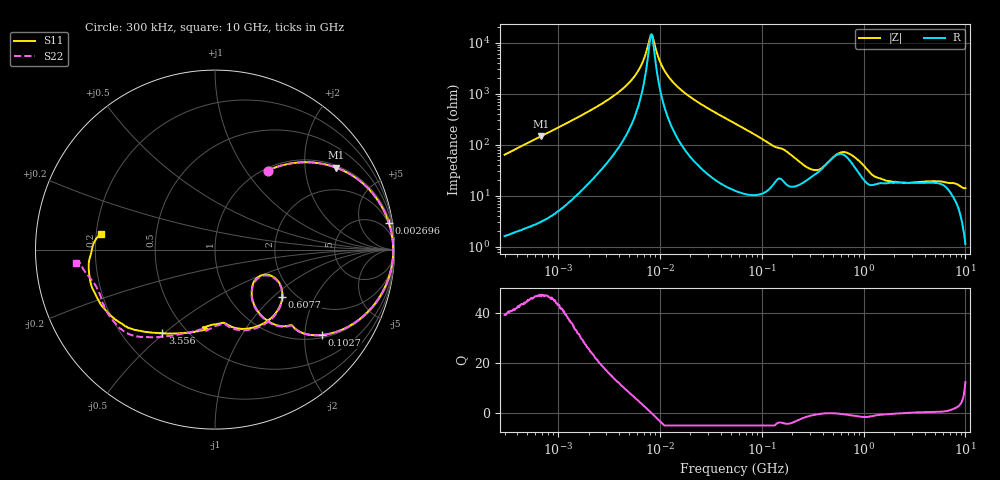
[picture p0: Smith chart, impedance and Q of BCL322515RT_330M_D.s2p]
! S-Parameter Data Generated by TDK Corporation
! Copyright(C) 2024 TDK Corporation.
! All Rights Reserved.
! TDK P/N: BCL322515RT-330M-D (SMD / SMT Inductor (Coil))
! Property: L=33uH at 1MHz
! Size(LxWxT): 3.2x2.5x1.5mm
! Model Type: s2p (Touchstone File Format Version 1.0)
! Frequency: DC=Yes Start=0.3MHz Stop=10000MHz 802points Log-sweep
! Model Generated on May 28, 2024
! Terms and conditions regarding TDK Simulation Models:
! 1)This simulation model is being provided solely for informational
!  purposes. Please refer to the specifications of the products in
!  terms of detailed characteristics of such products.
! 2)In no event shall TDK Corporation of any of its subsidiaries be
!  liable for any loss or damage arising, directly or indirectly,
!  from any information contained in this simulation model, including,
!  but not limited to loss or damages arising from any inaccuracies,
!  omissions or errors in connection with such information.
! 3)Any and all copyrights on this simulation model are owned by
!  TDK Corporation.  Duplication or redistribution of this simulation
!  model without prior written permission from TDK Corporation
!  is prohibited.
! 4)This simulation model is subject to any modification or change
!  without any prior notice.
! 5)Neither TDK Corporation nor any of its subsidiaries shall make any
!  warranty, express or implied, including but not limited to the
!  correctness, implied warranties of merchantability and fitness for
!  a particular purpose with respect to this simulation models.
! 6)The use of this simulation model shall be deemed to have consented
!  to the terms and conditions hereof.
! Port Assignments:
!  1 ---@@@--- 2
! Applicable Conditions:
!  Temperature = 25 degC
!  DC Bias Current = 0 A
!  Small Signal Operation
# Hz S MA R 50
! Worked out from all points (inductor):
!   801 points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, 300 kHz to 10 GHz, reference 50 ohm
!   read as one part in series: L = 33.7 uH near 318.3 kHz
!   highest Q = 47.1 at 680.6 kHz (marker M1), where L = 33.9 uH
!   self-resonance near 8.247 MHz
!   S11 on the Smith chart (normalised r, x): 300 kHz: 1.04, +1.27; 2.696 MHz: 2, +13; 102.7 MHz: 1.08, -2.43; 607.7 MHz: 1.72, -1.14; 3.556 GHz: 0.37, -0.49; 10 GHz: 0.22, +0.06
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300000  0.5287 56.3  0.8348 -32.2  0.8351 -32.1  0.529 56.4
680647  0.8148 34.1  0.5626 -54.7  0.5629 -54.6  0.8146 34.1
1713600  0.9585 14.6  0.2541 -73.4  0.2542 -73.4  0.9585 14.6
2695816  0.9798 8.8  0.1548 -78.2  0.1548 -78.2  0.9798 8.8
5784355  0.9919 2.2  0.04268 -78.0  0.04274 -78.1  0.992 2.2
6813581  0.9927 1.1  0.02364 -71.8  0.02366 -71.8  0.9928 1.1
8128066  0.9931 -0.1  0.007158 -18.1  0.007229 -17.6  0.9932 -0.1
8603105  0.9931 -0.5  0.008183 32.3  0.008111 32.0  0.9932 -0.5
9671944  0.993 -1.3  0.01922 68.0  0.01923 68.0  0.9931 -1.3
1.191229e7  0.9922 -2.8  0.04351 78.2  0.04351 78.2  0.9924 -2.8
1.626666e7  0.9892 -5.3  0.08432 79.8  0.08434 79.8  0.9894 -5.3
5.477226e7  0.9195 -22.1  0.3516 65.1  0.3516 65.1  0.9195 -22.2
1.026642e8  0.7608 -38.7  0.5868 46.3  0.587 46.3  0.7611 -38.8
1.900804e8  0.5236 -52.1  0.7461 25.2  0.7463 25.3  0.5236 -52.4
3.126428e8  0.3033 -47.4  0.7833 4.7  0.7835 4.7  0.3021 -46.9
4.448526e8  0.3228 -25.7  0.6849 -6.4  0.6851 -6.4  0.328 -26.2
6.076905e8  0.4573 -34.9  0.5782 -2.9  0.5784 -2.9  0.4616 -35.6
9.101824e8  0.4818 -64.9  0.6965 1.1  0.6967 1.1  0.4887 -65.6
1.767019e9  0.4219 -93.3  0.7513 -23.7  0.7514 -23.7  0.4324 -91.6
3.556288e9  0.551 -122.2  0.6373 -52.6  0.6375 -52.7  0.5659 -120.9
6.495326e9  0.6814 -146.0  0.4888 -79.5  0.4887 -79.7  0.6935 -146.7
1e10  0.6416 172.3  0.3363 -111.9  0.3361 -112.0  0.7756 -174.7
